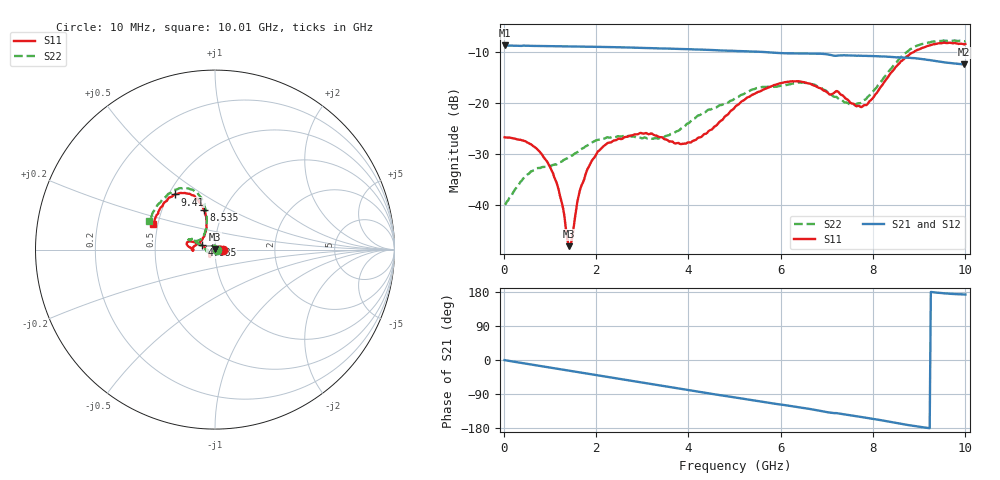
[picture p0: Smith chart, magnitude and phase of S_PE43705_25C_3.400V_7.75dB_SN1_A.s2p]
! Device ID: PE43705
! Serial: 1
! Insertion: A
! Impedance: 50 ohm
! Temp: 25C
! VDD: 3.400V
! Attenuation Step: 7.75dB
#  Hz  S  RI  R  50
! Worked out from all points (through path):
!   401 points, 10 MHz to 10.01 GHz, reference 50 ohm
!   highest |S21| = -8.82 dB at 10 MHz (marker M1); lowest = -12.5 dB at 9.985 GHz (marker M2)
!   group delay of S21, straight-line fit = 53.4 ps
!   lowest |S11| = -48.1 dB at 1.41 GHz (marker M3), VSWR 1.01, Z = 49.8 + j0.341 ohm
!   |S11| at or under -10 dB: start of sweep to 8.903 GHz
!   |S22| runs from -39.9 to -7.8 dB; largest |S21 - S12| = 0.0033
!   S11 on the Smith chart (normalised r, x): 10 MHz: 1.10, +0.00; 4.885 GHz: 0.86, +0.05; 8.535 GHz: 0.80, +0.38; 9.41 GHz: 0.54, +0.39; 10.01 GHz: 0.47, +0.16
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1e7  0.0457 3.75e-05  0.3624 -0.0018  0.3628 -0.00155  0.0101 0.000298
4.6e8  0.0393 0.0141  0.3552 -0.0596  0.3553 -0.0589  0.00687 0.0178
9.35e8  0.0208 0.016  0.3379 -0.1167  0.3381 -0.1164  -0.00759 0.0227
1.185e9  0.00888 0.0107  0.3255 -0.1447  0.3254 -0.1444  -0.0172 0.0191
1.41e9  -0.0019 0.00342  0.3121 -0.1691  0.3123 -0.169  -0.0257 0.0142
1.46e9  -0.00422 0.00108  0.3089 -0.1743  0.3091 -0.1743  -0.0276 0.0124
1.685e9  -0.0135 -0.00785  0.2933 -0.1971  0.2934 -0.1969  -0.0348 0.00575
1.885e9  -0.0208 -0.0155  0.278 -0.2161  0.2782 -0.2159  -0.0402 -5.29e-05
2.21e9  -0.0266 -0.0284  0.2504 -0.2445  0.2505 -0.2445  -0.0444 -0.00826
3.36e9  -0.0282 -0.0365  0.1329 -0.3125  0.1332 -0.3121  -0.044 -0.00689
4.06e9  -0.0395 -0.0106  0.0544 -0.3277  0.0548 -0.3275  -0.0656 0.0122
4.885e9  -0.0749 0.027  -0.0365 -0.3197  -0.0357 -0.3198  -0.0957 0.0354
5.01e9  -0.0845 0.0318  -0.0498 -0.3166  -0.0495 -0.3168  -0.1029 0.0394
5.96e9  -0.1463 0.0453  -0.1377 -0.273  -0.1368 -0.2731  -0.133 0.0565
6.685e9  -0.1484 0.0175  -0.1954 -0.2301  -0.1953 -0.2298  -0.1404 0.0538
7.435e9  -0.1045 0.0269  -0.2361 -0.1686  -0.2354 -0.1694  -0.0819 0.0572
7.76e9  -0.0696 0.0577  -0.2503 -0.1403  -0.2498 -0.1414  -0.0609 0.0814
8.36e9  -0.0485 0.1799  -0.2683 -0.0827  -0.2677 -0.0838  -0.0489 0.2001
8.535e9  -0.0638 0.2233  -0.2701 -0.0635  -0.2694 -0.0665  -0.0604 0.2472
9.41e9  -0.2225 0.3074  -0.2535 0.0112  -0.2528 0.0108  -0.229 0.3314
9.985e9  -0.3374 0.1546  -0.2346 0.0288  -0.2355 0.0288  -0.3582 0.1731
1.001e10  -0.3451 0.1454  -0.2354 0.0296  -0.2366 0.0291  -0.3661 0.1616
